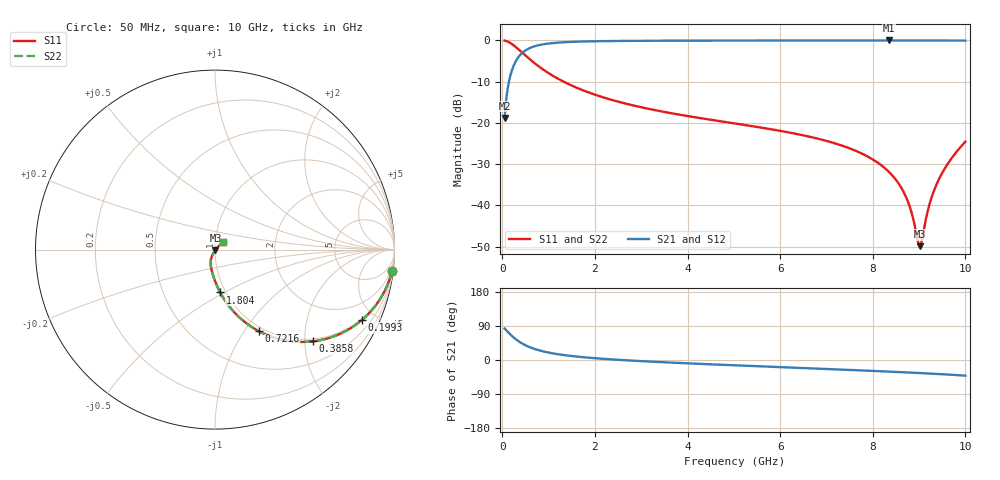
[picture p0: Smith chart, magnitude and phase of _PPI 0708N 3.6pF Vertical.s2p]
! S-Parameter data specifications (vertical orientation):
! Substrate: 40-mil Rogers 3003C, Substrate thickness, H=1.016mm, Dielectric constant, Er=3, Conductor thickness, T_mtl=0.043mm, Loss Tangent, Tand=0.003
! PCB Mounting Pad Footprint: Pad width, PadW=2.54mm , Pad length, PadL=0.51mm , Pad gap, PadG (edge-to-edge)=0.71mm , Reference planes=1.73mm apart
! Created Tue Jan 16 08:45:11 2018
# GHz S MA R 50
! 2 Port Network Data from SP1.SP block
! freq  magS11  angS11  magS21  angS21  magS12  angS12  magS22  angS22
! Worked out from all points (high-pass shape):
!   801 points, 50 MHz to 10 GHz, reference 50 ohm
!   highest |S21| = -0.03 dB at 8.346 GHz (marker M1); lowest = -18.8 dB at 50 MHz (marker M2)
!   |S21| within 3 dB of the highest: 432 MHz to end of sweep
!   lowest |S11| = -49.9 dB at 9.017 GHz (marker M3), VSWR 1.01, Z = 50.3 - j0.182 ohm
!   |S11| at or under -10 dB: 1.322 GHz to end of sweep
!   |S22| runs from -49.9 to -0.1 dB; largest |S21 - S12| = 0
!   S11 on the Smith chart (normalised r, x): 50 MHz: 1, -17; 199.2 MHz: 0.94, -4.22; 385.8 MHz: 0.94, -2.18; 721.6 MHz: 0.94, -1.17; 1.804 GHz: 0.94, -0.48; 10 GHz: 1.09, +0.09
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0.05  0.9934 -6.8  0.1149 83.2  0.1149 83.2  0.9934 -6.8
0.1370625  0.9532 -18.1  0.3021 71.9  0.3021 71.9  0.9532 -18.1
0.19925  0.9082 -25.5  0.4183 64.5  0.4183 64.5  0.9082 -25.5
0.3858125  0.7466 -43.2  0.6649 46.8  0.6649 46.8  0.7466 -43.2
0.721625  0.5161 -61.7  0.856 28.2  0.856 28.2  0.5161 -61.7
1.107187  0.368 -72.7  0.9292 17.2  0.9292 17.2  0.368 -72.7
1.716625  0.2515 -82.1  0.9671 7.7  0.9671 7.7  0.2515 -82.1
1.803688  0.2408 -83.1  0.9698 6.8  0.9698 6.8  0.2408 -83.1
3.370812  0.1401 -94.9  0.989 -5.3  0.989 -5.3  0.1401 -94.9
5.025  0.09833 -103.3  0.9937 -14.1  0.9937 -14.1  0.09833 -103.3
6.691625  0.06688 -110.7  0.9958 -22.1  0.9958 -22.1  0.06688 -110.7
7.699063  0.04421 -114.4  0.9966 -27.2  0.9966 -27.2  0.04421 -114.4
8.345812  0.02558 -114.9  0.9968 -30.6  0.9968 -30.6  0.02558 -114.9
8.718937  0.01261 -109.6  0.9967 -32.7  0.9967 -32.7  0.01261 -109.6
8.843312  0.007966 -101.3  0.9966 -33.4  0.9966 -33.4  0.007966 -101.3
8.967688  0.003824 -68.8  0.9965 -34.1  0.9965 -34.1  0.003824 -68.8
9.017437  0.00321 -34.4  0.9964 -34.4  0.9964 -34.4  0.00321 -34.4
9.067187  0.003966 -0.5  0.9964 -34.7  0.9964 -34.7  0.003966 -0.5
9.228875  0.01051 34.7  0.9961 -35.8  0.9961 -35.8  0.01051 34.7
9.390562  0.0187 41.4  0.9956 -36.8  0.9956 -36.8  0.0187 41.4
9.664188  0.03481 44.0  0.9946 -38.7  0.9946 -38.7  0.03481 44.0
10  0.05929 43.4  0.9924 -41.3  0.9924 -41.3  0.05929 43.4
